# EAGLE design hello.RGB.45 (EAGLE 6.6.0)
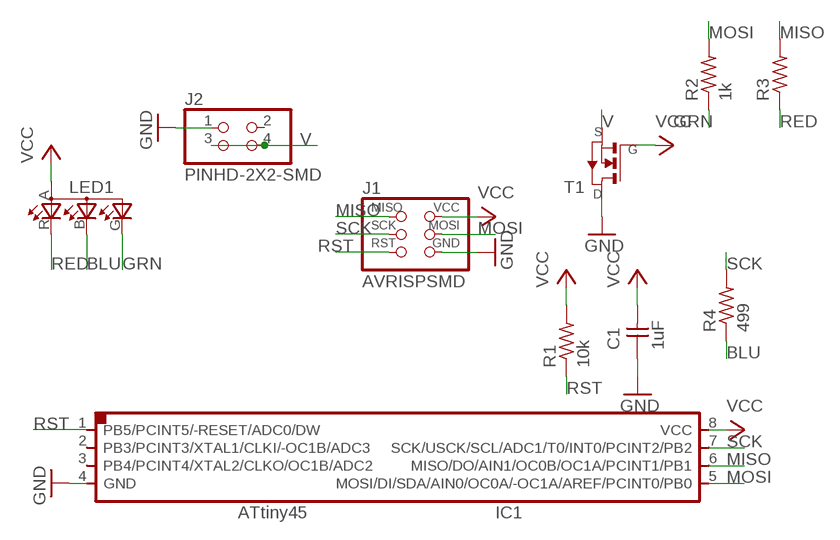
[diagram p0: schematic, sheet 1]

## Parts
C1  1uF  CAP-UNPOLARIZEDFAB  [C1206FAB]
IC1  ATTINY45SI  [SOIC8]
J1  AVRISPSMD  [2X03SMD]
J2  PINHD-2X2-SMD  [2X02SMD]
LED1  LEDRGBOLD  [P-LCC-4-3]
R1  10k  RES-US1206FAB  [R1206FAB]
R2  1k  RES-US1206FAB  [R1206FAB]
R3  RES-US1206FAB  [R1206FAB]
R4  499  RES-US1206FAB  [R1206FAB]
T1  NMOSFETSOT23  [SOT-23]

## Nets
BLU: LED1.B(CBLUE) R4.1
GND: C1.1 IC1.4(GND) J1.6(GND) J2.1 T1.1(D)
GRN: LED1.G(CGREEN) R2.1
MISO: IC1.6(MISO/DO/AIN1/OC0B/OC1A/PCINT1/PB1) J1.1(MISO) R3.2
MOSI: IC1.5(MOSI/DI/SDA/AIN0/OC0A/-OC1A/AREF/PCINT0/PB0) J1.4(MOSI) R2.2
RED: LED1.R(CRED) R3.1
RST: IC1.1(PB5/PCINT5/-RESET/ADC0/DW) J1.5(RST) R1.1
SCK: IC1.7(SCK/USCK/SCL/ADC1/T0/INT0/PCINT2/PB2) J1.3(SCK) R4.2
V: J2.3 J2.4 T1.2(S)
VCC: C1.2 IC1.8(VCC) J1.2(VCC) LED1.A(A2) R1.2 T1.3(G)
Unconnected: IC1.2(PB3/PCINT3/XTAL1/CLKI/-OC1B/ADC3) IC1.3(PB4/PCINT4/XTAL2/CLKO/OC1B/ADC2) J2.2

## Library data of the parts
C1 = fab:CAP-UNPOLARIZED
IC1 = fab:ATTINY45
J1 = fab:AVRISP
J2 = fab:PINHD-2X2-SMD
LED1 = fab:LEDRGBOLD: OSRAM Hyper Multi TOPLED® Hyper-Bright LED LATB T686 Source: http://www.osram.convergy.de/
R1-R4 = fab:RES-US: Resistor (US Symbol)
T1 = fab:NMOSFET: MOS FET

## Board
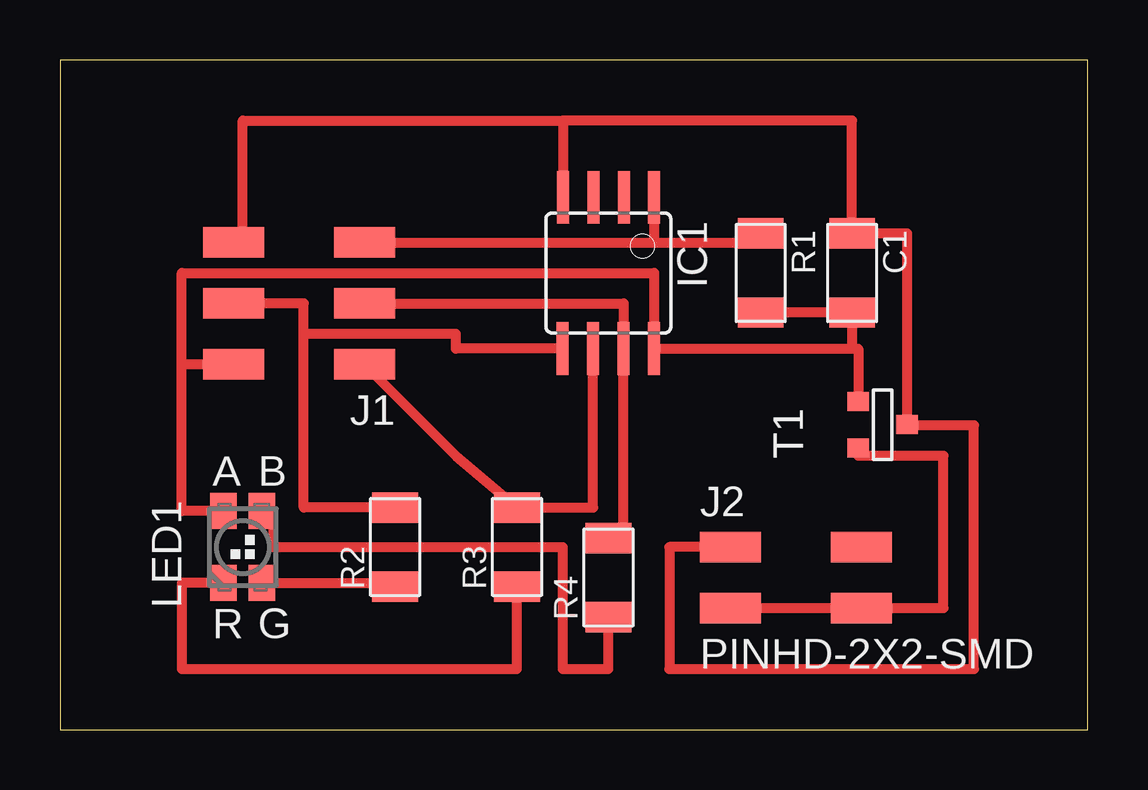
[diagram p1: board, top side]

Size 42.85 x 27.93 mm. Coordinates in mm from the lower left corner, seen from the top.
Outline: 0,0 42.85,0 42.85,27.93 0,27.93 0,0
Copper layers (1*16): Top 0.035mm / dielectric 1.5mm / Bottom 0.035mm
Design rules "fabmodule": minimum track width 10mil, minimum drill 0.4mm, track to track 0.42mm, track to pad 0.42mm, pad to pad 0.42mm, via to via 0.42mm, smd to smd 0.42mm, copper to edge 40mil, drill to drill 0.8mm, minimum pad ring 10mil, minimum via ring 8mil, stop-mask expansion 4mil, vias tented up to drill 0mil, thermal gap 10mil

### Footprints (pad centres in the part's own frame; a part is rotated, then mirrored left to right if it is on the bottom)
C1206FAB = smd 1.27 x 1.905: 1 -1.651,0; 2 1.651,0
SOIC8 = smd 0.5 x 2.2: 1 -1.905,-3.154; 2 -0.645,-3.154; 3 0.625,-3.154; 4 1.895,-3.154; 5 1.905,3.154; 6 0.635,3.154; 7 -0.635,3.154; 8 -1.905,3.154
2X03SMD = smd 2.54 x 1.27: 1 -2.54,2.54; 2 2.92,2.54; 3 -2.54,0; 4 2.92,0; 5 -2.54,-2.54; 6 2.92,-2.54
2X02SMD = smd 2.54 x 1.27: 1 -2.54,1.27; 2 2.92,1.27; 3 -2.54,-1.27; 4 2.92,-1.27
P-LCC-4-3 = smd 1.1 x 1.5: A -0.8,1.5; B 0.8,1.5; G 0.8,-1.5; R -0.8,-1.5
R1206FAB = smd 1.27 x 1.905: 1 -1.651,0; 2 1.651,0
SOT-23 = smd 0.787 x 0.889: 1 0.025,-1.016; 2 -0.94,1.016; 3 0.991,1.016

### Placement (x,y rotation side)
C1  33.02,19.05 270 top
IC1  22.86,19.05 180 top
J1  10.16,17.78 180 top
J2  30.48,6.35 0 top
LED1  7.62,7.62 0 top
R1  29.21,19.05 270 top
R2  13.97,7.62 90 top
R3  19.05,7.62 90 top
R4  22.86,6.35 90 top
T1  34.29,12.7 90 top

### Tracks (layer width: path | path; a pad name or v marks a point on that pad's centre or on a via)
BLU
  Top 0.406: LED1.B 8.89,9.12 8.89,7.62 20.95,7.62 20.95,2.54 22.86,2.54 R4.1
GND
  Top 0.406: J1.6 7.62,20.32 7.62,25.4 20.96,25.4 | 20.96,25.4 IC1.4 | 20.96,25.4 33.02,25.4 C1.1 35.31,20.7 T1.1 35.31,12.7 38.1,12.7 38.1,2.54 25.4,2.54 25.4,7.62 J2.1
GRN
  Top 0.406: LED1.G 13.97,6.12 R2.1
MISO
  Top 0.406: J1.1 16.51,11.43 R3.2 22.23,9.27 IC1.6
MOSI
  Top 0.406: IC1.5 16.51,15.9 16.51,16.51 10.16,16.51 | 10.16,16.51 10.16,17.78 J1.4 | R2.2 10.16,9.27 10.16,16.51
RED
  Top 0.406: LED1.R 5.08,6.12 5.08,2.54 19.05,2.54 R3.1
RST
  Top 0.406: J1.5 24.77,20.32 | 24.77,20.32 29.21,20.32 R1.1 | IC1.1 24.77,20.32
SCK
  Top 0.406: J1.3 23.5,17.78 IC1.7 23.5,8 R4.2
V
  Top 0.406: J2.3 J2.4 36.83,5.08 36.83,11.43 33.27,11.43 T1.2
VCC
  Top 0.406: R1.2 C1.2 33.02,15.9 | 33.02,15.9 IC1.8 24.77,19.05 5.08,19.05 5.08,15.24 | 33.02,15.9 33.27,15.9 T1.3 | LED1.A 5.08,9.12 5.08,15.24 | J1.2 5.08,15.24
